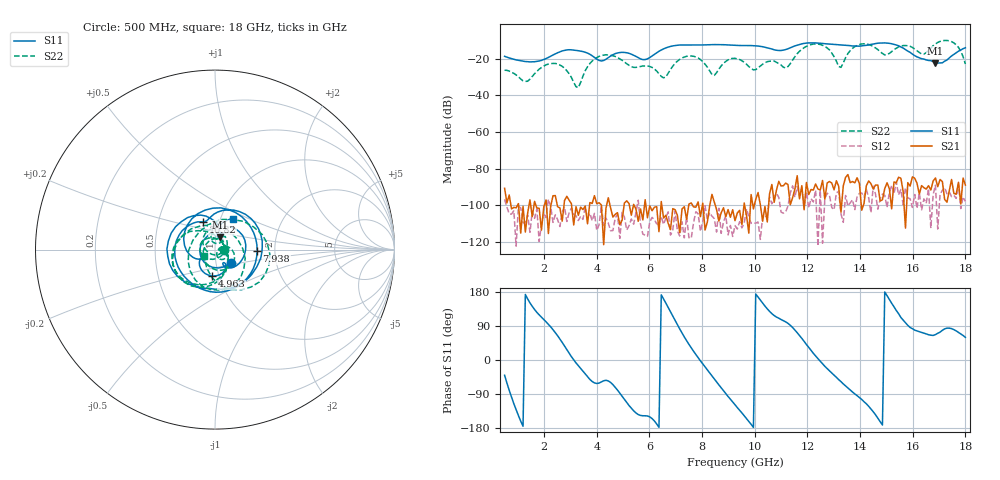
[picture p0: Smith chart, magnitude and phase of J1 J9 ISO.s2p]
!Agilent Technologies,N5230A,MY45001360,A.07.50.67
!Agilent N5230A: A.07.50.67
!Date: Tuesday, April 16, 2024 17:52:33
!Correction: S11(Full 2 Port(1,2))
!S21(Full 2 Port(1,2))
!S12(Full 2 Port(1,2))
!S22(Full 2 Port(1,2))
!S2P File: Measurements: S11, S21, S12, S22:
# Hz S  dB  R 50
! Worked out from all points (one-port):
!   201 points, 500 MHz to 18 GHz, reference 50 ohm
!   lowest |S11| = -22.5 dB at 16.86 GHz (marker M1), VSWR 1.16, Z = 52.5 + j7.26 ohm
!   |S11| at or under -10 dB: start of sweep to end of sweep
!   S11 on the Smith chart (normalised r, x): 500 MHz: 1.18, -0.18; 4.963 GHz: 0.93, -0.28; 7.938 GHz: 1.61, -0.03; 10.82 GHz: 0.84, +0.27; 18 GHz: 1.14, +0.41
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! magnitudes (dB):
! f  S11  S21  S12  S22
! 500 MHz  -18.7  -90.6  -96.6  -26.3
! 1.375 GHz  -21.7  -104.2  -105.3  -32.3
! 2.513 GHz  -16.8  -100.7  -107.7  -22.9
! 3.3 GHz  -15.7  -105.4  -108.2  -35.8
! 3.475 GHz  -16.2  -102.2  -107.6  -29.6
! 4.088 GHz  -21.0  -98.5  -110.5  -18.8
! 4.963 GHz  -16.6  -108.0  -103.7  -20.9
! 6.362 GHz  -16.0  -114.3  -110.4  -28.2
! 7.325 GHz  -12.5  -100.7  -117.7  -19.1
! 7.938 GHz  -12.6  -106.1  -114.1  -20.5
! 8.463 GHz  -12.4  -98.1  -107.2  -29.1
! 9.25 GHz  -12.7  -108.3  -111.0  -19.9
! 9.95 GHz  -13.0  -101.9  -109.7  -26.1
! 10.82 GHz  -15.4  -91.6  -93.3  -22.0
! 11.18 GHz  -15.1  -87.8  -103.5  -25.1
! 12.22 GHz  -11.4  -91.6  -98.1  -12.1
! 13.28 GHz  -12.5  -103.7  -104.5  -24.8
! 13.97 GHz  -13.2  -88.1  -93.5  -12.3
! 15.11 GHz  -11.7  -90.8  -92.9  -17.2
! 16.86 GHz  -22.5  -85.0  -88.9  -12.1
! 17.56 GHz  -17.7  -93.4  -94.4  -11.5
! 18 GHz  -14.1  -88.9  -97.8  -22.9
